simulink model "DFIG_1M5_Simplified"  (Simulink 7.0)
settings: Solver=ode45  SolverMode=SingleTasking  StartTime=0  StopTime=Tstop  FixedStep=0,000005  MaxStep=0.001  RelTol=1e-3  AbsTol=1e-6
InitFcn:
  | DFIG_init_simp
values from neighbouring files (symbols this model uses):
  gearbox = 75.7098    [DFIG_init_simp.m]    (also in DFIG_init_sw.m)
  ki_i = 0.003    [DFIG_init_simp.m]    (also in DFIG_init_sw.m)
  kp_i = 0.00003    (= 3e-05)    [DFIG_init_simp.m]    (also in DFIG_init_sw.m)
  L = 0.6e-3    (= 0.0006)    [DFIG_init_simp.m]    (also in DFIG_init_sw.m)
  R = 35    [DFIG_init_simp.m]    (also in DFIG_init_sw.m)
  TSR_opt = 8    [DFIG_init_simp.m]    (also in DFIG_init_sw.m)
  Tswitch = 0.2    [DFIG_init_simp.m]    (also in DFIG_init_sw.m)
  Vw1 = 10.5    [DFIG_init_simp.m]    (also in DFIG_init_sw.m)
  Vw2 = 8    [DFIG_init_simp.m]    (also in DFIG_init_sw.m)
  zp = 2    [DFIG_init_simp.m]    (also in DFIG_init_sw.m)
undefined symbols (not defined in the file or in its folder): plecsedit
libraries: plecslib x10, plecslib_extras x4, simulink x2

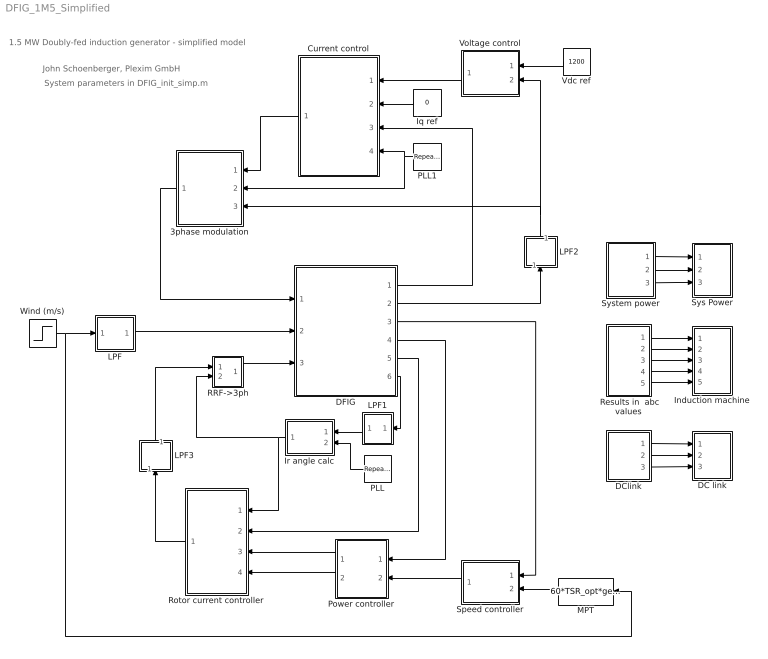
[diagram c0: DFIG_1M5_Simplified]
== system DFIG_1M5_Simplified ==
  note: John Schoenberger, Plexim GmbH
  note: 1.5 MW Doubly-fed induction generator - simplified model
  note: System parameters in DFIG_init_simp.m
  " Results in  abc values" : Subsystem
  3phase modulation : Subsystem  Orientation=left
  Current control : Subsystem  Orientation=left
  DC link : Subsystem  LoadFcn=plecsedit('sl', 300);  StartFcn=plecsedit('sl', 308);  StopFcn=plecsedit('sl', 309);  mask{Settings=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}
      mask init:
      | plecsedit('sl', 315);
  DClink : Subsystem
  DFIG : Subsystem  LoadFcn=plecsedit('sl', 200);  InitFcn=plecsedit('sl', 214);  StartFcn=plecsedit('sl', 208);  StopFcn=plecsedit('sl', 209);
  Induction machine : Subsystem  LoadFcn=plecsedit('sl', 300);  StartFcn=plecsedit('sl', 308);  StopFcn=plecsedit('sl', 309);  mask{Settings=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}
      mask init:
      | plecsedit('sl', 315);
  Iq ref : Constant  Orientation=left  Value=0  OutDataType=sfix(16)  OutScaling=2^0
  Ir angle calc : Subsystem  Orientation=left
  LPF : Subsystem  mask{tau=0.2, y0=Vw1}
      mask prompts: tau "Time constant"; y0 "Initial output"
  LPF1 : Subsystem  Orientation=left  mask(Low-pass filter){tau=1e-4, y0=0}
      mask prompts: tau "Time constant"; y0 "Initial output"
      mask help: First order low pass filter, used in the same way as a memory block to break an algebraic loop. Provides a more deterministic output with a variable-step simulation.
  LPF2 : Subsystem  Orientation=up  mask(Low-pass filter){tau=1e-4, y0=0}
      mask prompts: tau "Time constant"; y0 "Initial output"
      mask help: First order low pass filter, used in the same way as a memory block to break an algebraic loop. Provides a more deterministic output with a variable-step simulation.
  LPF3 : Subsystem  Orientation=up  mask(Low-pass filter){tau=0.5e-4, y0=[0 0]}
      mask prompts: tau "Time constant"; y0 "Initial output"
      mask help: First order low pass filter, used in the same way as a memory block to break an algebraic loop. Provides a more deterministic output with a variable-step simulation.
  MPT : Fcn  Orientation=left  Expr=60*TSR_opt*gearbox*u(1)/(2*pi*R)
  PLL : simulink/Sources/Repeating Sequence  Orientation=left  SystemSampleTime=-1  rep_seq_t=[0 0.02]  rep_seq_y=[-pi/2 3/2*pi]
  PLL1 : simulink/Sources/Repeating Sequence  Orientation=left  SystemSampleTime=-1  rep_seq_t=[0 0.02]  rep_seq_y=[-pi/2 3/2*pi]
  Power controller : Subsystem  Orientation=left
  RRF->3ph : Subsystem  AncestorBlock=plecslib_extras/Transformations/RRF->3ph
  Rotor current controller : Subsystem  Orientation=left
  Speed controller : Subsystem  Orientation=left
  Sys Power : Subsystem  LoadFcn=plecsedit('sl', 300);  StartFcn=plecsedit('sl', 308);  StopFcn=plecsedit('sl', 309);  mask{Settings=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}
      mask init:
      | plecsedit('sl', 315);
  System power : Subsystem
  Vdc ref : Constant  Orientation=left  Value=1200  OutDataType=sfix(16)  OutScaling=2^0
  Voltage control : Subsystem  Orientation=left
  Wind (m/s) : Step  Time=Tswitch  Before=Vw1  After=Vw2  SampleTime=0
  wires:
  RRF->3ph/1(abc) -> DFIG/3(m2)
  DFIG/5(Ir2) -> Rotor current controller/2(Ir2)
  DFIG/6(th r) -> LPF1/1(x)
  Ir angle calc/1(th Ir) -> Rotor current controller/1(theta), RRF->3ph/2(phi)
  " Results in  abc values"/1(Irabc) -> Induction machine/1(1)
  " Results in  abc values"/2(Isabc) -> Induction machine/2(2)
  " Results in  abc values"/3(Vrabc) -> Induction machine/3(3)
  " Results in  abc values"/4(speed) -> Induction machine/4(4)
  " Results in  abc values"/5(Torque) -> Induction machine/5(5)
  DClink/1(Idc in) -> DC link/1(1)
  DClink/2(Vdc) -> DC link/2(2)
  DClink/3(Pdc in) -> DC link/3(3)
  Wind (m/s)/1 -> LPF/1(Vw), MPT/1
  LPF/1(Vw') -> DFIG/2(Vwind)
  Power controller/1(Irq*) -> Rotor current controller/3(Irq*)
  Power controller/2(Ird*) -> Rotor current controller/4(Ird*)
  PLL/1 -> Ir angle calc/2(th 50Hz)
  DFIG/1(Ir1) -> Current control/3(Ir1)
  DFIG/2(Vdc) -> LPF2/1(x)
  System power/1(Stator PQ) -> Sys Power/1(1)
  System power/2(Rotor PQ) -> Sys Power/2(2)
  System power/3(Sys PQ) -> Sys Power/3(3)
  Speed controller/1(P*) -> Power controller/2(P*)
  DFIG/3(rpm) -> Speed controller/1(rpm)
  DFIG/4(P,Q) -> Power controller/1(S)
  MPT/1 -> Speed controller/2(rpm*)
  Voltage control/1(Id*) -> Current control/1(Id*)
  Vdc ref/1 -> Voltage control/1(Vdc*)
  LPF2/1(x') -> 3phase modulation/3(Vdc), Voltage control/2(Vdc)
  Iq ref/1 -> Current control/2(Iq*)
  Current control/1(Vdq*) -> 3phase modulation/1(Vdq*)
  3phase modulation/1(m1) -> DFIG/1(m1)
  PLL1/1 -> 3phase modulation/2(theta), Current control/4(theta)
  LPF1/1(x') -> Ir angle calc/1(th r)
  Rotor current controller/1(Vr dq*) -> LPF3/1(x)
  LPF3/1(x') -> RRF->3ph/1(dq)

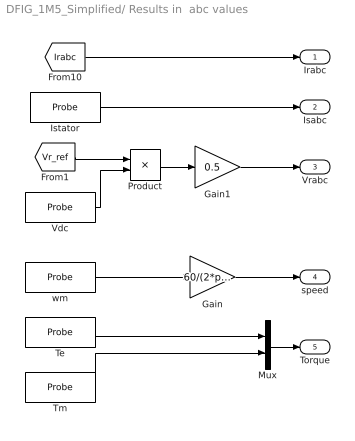
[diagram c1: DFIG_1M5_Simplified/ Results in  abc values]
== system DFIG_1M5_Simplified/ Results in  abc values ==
  Gain : Gain  Gain=60/(2*pi)  ParameterDataType=sfix(16)  ParameterScaling=2^0  OutDataType=sfix(16)  OutScaling=2^0
  Gain1 : Gain  Gain=0.5  ParameterDataType=sfix(16)  ParameterScaling=2^0  OutDataType=sfix(16)  OutScaling=2^0
  Istator : plecslib/Probe  SystemSampleTime=-1  tagno=3
  Mux : Mux  Inputs=2
  Product : Product  OutDataType=sfix(16)  OutScaling=2^0
  Te : plecslib/Probe  SystemSampleTime=-1  tagno=1
  Tm : plecslib/Probe  SystemSampleTime=-1  tagno=5
  Vdc : plecslib/Probe  SystemSampleTime=-1  tagno=4
  wm : plecslib/Probe  SystemSampleTime=-1  tagno=2
  Irabc : Outport
  Isabc : Outport  Port=2
  Vrabc : Outport  Port=3
  speed : Outport  Port=4
  Torque : Outport  Port=5
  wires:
  Gain/1 -> speed/1
  Istator/1 -> Isabc/1
  [Irabc] -> Irabc/1
  Product/1 -> Gain1/1
  Te/1 -> Mux/1
  Tm/1 -> Mux/2
  Mux/1 -> Torque/1
  wm/1 -> Gain/1
  [Vr_ref] -> Product/1
  Vdc/1 -> Product/2
  Gain1/1 -> Vrabc/1

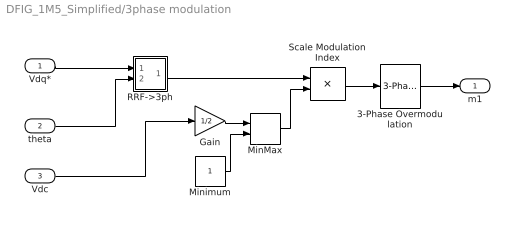
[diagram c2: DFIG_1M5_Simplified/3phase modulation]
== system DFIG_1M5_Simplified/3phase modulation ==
  Vdq* : Inport  OutDataType=sfix(16)  OutScaling=2^0
  theta : Inport  Port=2  OutDataType=sfix(16)  OutScaling=2^0
  Vdc : Inport  Port=3  OutDataType=sfix(16)  OutScaling=2^0
  3-Phase Overmodulation : plecslib_extras/Modulators/3-Phase Overmodulation  SystemSampleTime=-1
  Gain : Gain  Gain=1/2  ParameterDataType=sfix(16)  ParameterScaling=2^0  OutDataType=sfix(16)  OutScaling=2^0
  MinMax : MinMax  Function=max  Inputs=2  OutDataType=sfix(16)  OutScaling=2^0
  Minimum : Constant  OutDataType=sfix(16)  OutScaling=2^0
  RRF->3ph : Subsystem
  Scale Modulation Index : Product  Inputs=*/  OutDataType=sfix(16)  OutScaling=2^0
  m1 : Outport  OutDataType=sfix(16)  OutScaling=2^0
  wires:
  theta/1 -> RRF->3ph/2(phi)
  3-Phase Overmodulation/1 -> m1/1
  Gain/1 -> MinMax/1
  Minimum/1 -> MinMax/2
  MinMax/1 -> Scale Modulation Index/2
  Vdc/1 -> Gain/1
  Scale Modulation Index/1 -> 3-Phase Overmodulation/1
  RRF->3ph/1(abc) -> Scale Modulation Index/1
  Vdq*/1 -> RRF->3ph/1(dq)

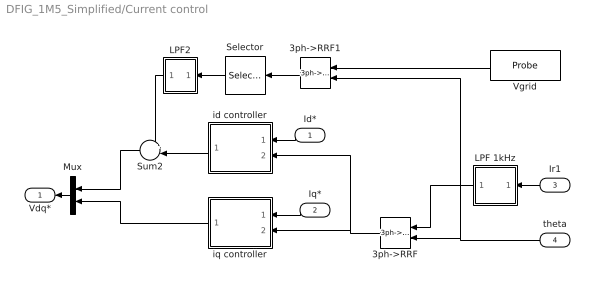
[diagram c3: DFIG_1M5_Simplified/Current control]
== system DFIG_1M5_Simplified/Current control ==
  Id* : Inport  Orientation=left
  Iq* : Inport  Orientation=left  Port=2
  Ir1 : Inport  Orientation=left  Port=3  OutDataType=sfix(16)  OutScaling=2^0
  theta : Inport  Orientation=left  Port=4  OutDataType=sfix(16)  OutScaling=2^0
  3ph->RRF : plecslib_extras/Transformations/3ph->RRF  Orientation=left  SystemSampleTime=-1
  3ph->RRF1 : plecslib_extras/Transformations/3ph->RRF  Orientation=left  SystemSampleTime=-1
  LPF 1kHz : Subsystem  Orientation=left  mask{tau=1.6e-4, y0=0}
      mask prompts: tau "Time constant"; y0 "Initial output"
  LPF2 : Subsystem  Orientation=left  mask(Low-pass filter){tau=1e-4, y0=0}
      mask prompts: tau "Time constant"; y0 "Initial output"
      mask help: First order low pass filter, used in the same way as a memory block to break an algebraic loop. Provides a more deterministic output with a variable-step simulation.
  Mux : Mux  Orientation=left  Inputs=2
  Selector : Selector  Orientation=left  InputPortWidth=2  IndexOptions=Index vector (dialog)  Indices=1  OutputSizes=1
  Sum2 : Sum  Orientation=left  Inputs=+-|  OutDataType=sfix(16)  OutScaling=2^0
  Vgrid : plecslib/Probe  Orientation=left  SystemSampleTime=-1  tagno=6
  id controller : Subsystem  Orientation=left
  iq controller : Subsystem  Orientation=left
  Vdq* : Outport  Orientation=left
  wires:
  iq controller/1(Vq*) -> Mux/2
  Sum2/1 -> Mux/1
  Mux/1 -> Vdq*/1
  Vgrid/1 -> 3ph->RRF1/1
  Ir1/1 -> LPF 1kHz/1(I)
  theta/1 -> 3ph->RRF1/2, 3ph->RRF/2
  Iq*/1 -> iq controller/1(iq ref)
  Id*/1 -> id controller/1(id ref)
  3ph->RRF1/1 -> Selector/1
  3ph->RRF/1 -> id controller/2(i), iq controller/2(i)
  id controller/1(Vd*) -> Sum2/2
  LPF 1kHz/1(Ifilt) -> 3ph->RRF/1
  Selector/1 -> LPF2/1(x)
  LPF2/1(x') -> Sum2/1

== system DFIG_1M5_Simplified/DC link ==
  1 : Inport  OutDataType=sfix(16)  OutScaling=2^0
  2 : Inport  Port=2  OutDataType=sfix(16)  OutScaling=2^0
  3 : Inport  Port=3  OutDataType=sfix(16)  OutScaling=2^0
  " InputMux " : Subsystem
  " S-Function " : S-Function  FunctionName=plecsedit
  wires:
  " InputMux "/1(Out) -> " S-Function "/1
  1/1 -> " InputMux "/1(In1)
  2/1 -> " InputMux "/2(In2)
  3/1 -> " InputMux "/3(In3)

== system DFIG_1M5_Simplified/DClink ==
  DC current from grid converter : plecslib/Probe  SystemSampleTime=-1  tagno=14
  Product : Product  OutDataType=sfix(16)  OutScaling=2^0
  vdc : plecslib/Probe  SystemSampleTime=-1  tagno=15
  Idc in : Outport
  Vdc : Outport  Port=2
  Pdc in : Outport  Port=3
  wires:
  DC current from grid converter/1 -> Idc in/1, Product/1
  vdc/1 -> Vdc/1, Product/2
  Product/1 -> Pdc in/1

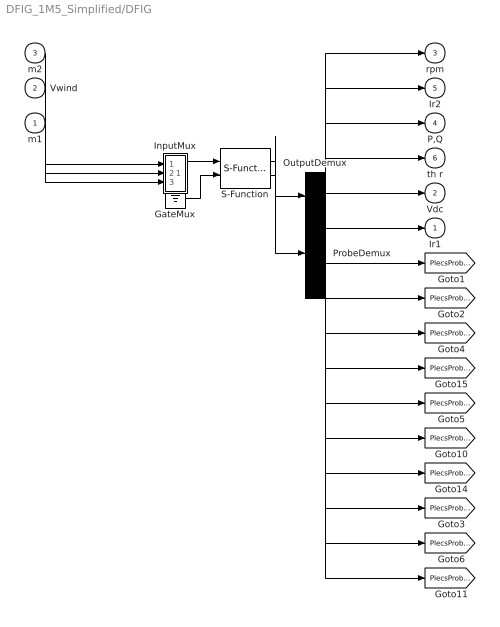
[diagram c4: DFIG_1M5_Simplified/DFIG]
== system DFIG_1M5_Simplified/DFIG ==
  m1 : Inport  PortDimensions=3  OutDataType=sfix(16)  OutScaling=2^0
  Vwind : Inport  Port=2  PortDimensions=1  OutDataType=sfix(16)  OutScaling=2^0
  m2 : Inport  Port=3  PortDimensions=3  OutDataType=sfix(16)  OutScaling=2^0
  " GateMux " : Ground
  " InputMux " : Subsystem
  " OutputDemux " : Demux  Outputs=[ 1 3 2 1 1 3 ]
  " ProbeDemux " : Demux  Outputs=[ 1 1 1 1 1 3 1 3 3 3 ]
  " S-Function " : S-Function  FunctionName=plecsedit
  Ir1 : Outport  PortDimensions=3  OutDataType=sfix(16)  OutScaling=2^0
  Vdc : Outport  Port=2  PortDimensions=1  OutDataType=sfix(16)  OutScaling=2^0
  rpm : Outport  Port=3  PortDimensions=1  OutDataType=sfix(16)  OutScaling=2^0
  P,Q : Outport  Port=4  PortDimensions=2
  Ir2 : Outport  Port=5  PortDimensions=3  OutDataType=sfix(16)  OutScaling=2^0
  th r : Outport  Port=6  PortDimensions=1  OutDataType=sfix(16)  OutScaling=2^0
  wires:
  " S-Function "/2 -> " ProbeDemux "/1
  " GateMux "/1 -> " S-Function "/2
  " InputMux "/1(Out) -> " S-Function "/1
  " S-Function "/1 -> " OutputDemux "/1
  m2/1 -> " InputMux "/1(In1)
  Vwind/1 -> " InputMux "/2(In2)
  m1/1 -> " InputMux "/3(In3)
  " OutputDemux "/1 -> rpm/1
  " OutputDemux "/2 -> Ir2/1
  " OutputDemux "/3 -> P,Q/1
  " OutputDemux "/4 -> th r/1
  " OutputDemux "/5 -> Vdc/1
  " OutputDemux "/6 -> Ir1/1
  " ProbeDemux "/1 -> [PlecsProbe1]
  " ProbeDemux "/2 -> [PlecsProbe2]
  " ProbeDemux "/3 -> [PlecsProbe4]
  " ProbeDemux "/4 -> [PlecsProbe15]
  " ProbeDemux "/5 -> [PlecsProbe5]
  " ProbeDemux "/6 -> [PlecsProbe10]
  " ProbeDemux "/7 -> [PlecsProbe14]
  " ProbeDemux "/8 -> [PlecsProbe3]
  " ProbeDemux "/9 -> [PlecsProbe6]
  " ProbeDemux "/10 -> [PlecsProbe11]

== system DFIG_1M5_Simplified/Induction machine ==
  1 : Inport  OutDataType=sfix(16)  OutScaling=2^0
  2 : Inport  Port=2  OutDataType=sfix(16)  OutScaling=2^0
  3 : Inport  Port=3  OutDataType=sfix(16)  OutScaling=2^0
  4 : Inport  Port=4  OutDataType=sfix(16)  OutScaling=2^0
  5 : Inport  Port=5  OutDataType=sfix(16)  OutScaling=2^0
  " InputMux " : Subsystem
  " S-Function " : S-Function  FunctionName=plecsedit
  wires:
  " InputMux "/1(Out) -> " S-Function "/1
  1/1 -> " InputMux "/1(In1)
  2/1 -> " InputMux "/2(In2)
  3/1 -> " InputMux "/3(In3)
  4/1 -> " InputMux "/4(In4)
  5/1 -> " InputMux "/5(In5)

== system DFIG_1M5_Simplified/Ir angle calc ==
  th r : Inport  OutDataType=sfix(16)  OutScaling=2^0
  th 50Hz : Inport  Port=2  OutDataType=sfix(16)  OutScaling=2^0
  Gain : Gain  Gain=zp  ParameterDataType=sfix(16)  ParameterScaling=2^0  OutDataType=sfix(16)  OutScaling=2^0
  Sum1 : Sum  Inputs=+-  OutDataType=sfix(16)  OutScaling=2^0
  th Ir : Outport
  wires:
  th r/1 -> Gain/1
  th 50Hz/1 -> Sum1/1
  Sum1/1 -> th Ir/1
  Gain/1 -> Sum1/2

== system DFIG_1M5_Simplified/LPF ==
  Vw : Inport  OutDataType=sfix(16)  OutScaling=2^0
  Gain : Gain  Gain=1/tau  ParameterDataType=sfix(16)  ParameterScaling=2^0  OutDataType=sfix(16)  OutScaling=2^0
  Integrator : Integrator  InitialCondition=y0
  Subtract : Sum  Inputs=+-  OutDataType=sfix(16)  OutScaling=2^-10
  Vw' : Outport  OutDataType=sfix(16)  OutScaling=2^0
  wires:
  Integrator/1 -> Vw'/1, Subtract/2
  Vw/1 -> Subtract/1
  Subtract/1 -> Gain/1
  Gain/1 -> Integrator/1

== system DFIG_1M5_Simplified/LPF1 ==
  x : Inport  OutDataType=sfix(16)  OutScaling=2^0
  Gain : Gain  Gain=1/tau  ParameterDataType=sfix(16)  ParameterScaling=2^0  OutDataType=sfix(16)  OutScaling=2^0
  Integrator : Integrator  InitialCondition=y0
  Subtract : Sum  Inputs=+-  OutDataType=sfix(16)  OutScaling=2^-10
  x' : Outport  OutDataType=sfix(16)  OutScaling=2^0
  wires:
  Integrator/1 -> x'/1, Subtract/2
  x/1 -> Subtract/1
  Subtract/1 -> Gain/1
  Gain/1 -> Integrator/1

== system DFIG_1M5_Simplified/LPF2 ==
  x : Inport  OutDataType=sfix(16)  OutScaling=2^0
  Gain : Gain  Gain=1/tau  ParameterDataType=sfix(16)  ParameterScaling=2^0  OutDataType=sfix(16)  OutScaling=2^0
  Integrator : Integrator  InitialCondition=y0
  Subtract : Sum  Inputs=+-  OutDataType=sfix(16)  OutScaling=2^-10
  x' : Outport  OutDataType=sfix(16)  OutScaling=2^0
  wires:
  Integrator/1 -> x'/1, Subtract/2
  x/1 -> Subtract/1
  Subtract/1 -> Gain/1
  Gain/1 -> Integrator/1

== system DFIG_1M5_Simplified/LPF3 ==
  x : Inport  OutDataType=sfix(16)  OutScaling=2^0
  Gain : Gain  Gain=1/tau  ParameterDataType=sfix(16)  ParameterScaling=2^0  OutDataType=sfix(16)  OutScaling=2^0
  Integrator : Integrator  InitialCondition=y0
  Subtract : Sum  Inputs=+-  OutDataType=sfix(16)  OutScaling=2^-10
  x' : Outport  OutDataType=sfix(16)  OutScaling=2^0
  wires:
  Integrator/1 -> x'/1, Subtract/2
  x/1 -> Subtract/1
  Subtract/1 -> Gain/1
  Gain/1 -> Integrator/1

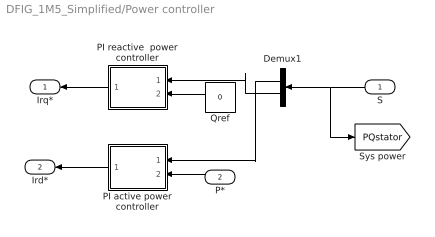
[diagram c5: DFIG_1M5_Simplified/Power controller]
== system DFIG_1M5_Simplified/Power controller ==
  S : Inport  Orientation=left  OutDataType=sfix(16)  OutScaling=2^0
  P* : Inport  Orientation=left  Port=2  OutDataType=sfix(16)  OutScaling=2^0
  Demux1 : Demux  Orientation=left  Outputs=2
  PI active power controller : Subsystem  Orientation=left
  PI reactive  power controller : Subsystem  Orientation=left
  Qref : Constant  Orientation=left  Value=0  OutDataType=sfix(16)  OutScaling=2^0
  Irq* : Outport  Orientation=left  OutDataType=sfix(16)  OutScaling=2^0
  Ird* : Outport  Orientation=left  Port=2  OutDataType=sfix(16)  OutScaling=2^0
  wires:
  Qref/1 -> PI reactive  power controller/2(Qref)
  PI reactive  power controller/1(Irqref) -> Irq*/1
  PI active power controller/1(Irdref) -> Ird*/1
  P*/1 -> PI active power controller/2(Pref)
  S/1 -> Demux1/1, [PQstator]
  Demux1/1 -> PI active power controller/1(P)
  Demux1/2 -> PI reactive  power controller/1(Q)

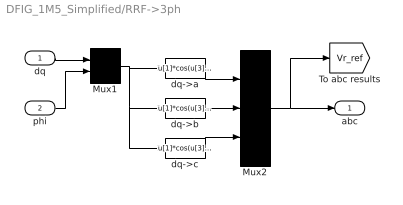
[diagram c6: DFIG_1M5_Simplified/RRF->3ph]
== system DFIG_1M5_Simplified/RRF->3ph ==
  dq : Inport  PortDimensions=2
  phi : Inport  Port=2  PortDimensions=1
  Mux1 : Mux  Inputs=2
  Mux2 : Mux  Inputs=3
  dq->a : Fcn  Expr=u[1]*cos(u[3])-u[2]*sin(u[3])
  dq->b : Fcn  Expr=u[1]*cos(u[3]-2*pi/3)-u[2]*sin(u[3]-2*pi/3)
  dq->c : Fcn  Expr=u[1]*cos(u[3]+2*pi/3)-u[2]*sin(u[3]+2*pi/3)
  abc : Outport
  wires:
  phi/1 -> Mux1/2
  dq/1 -> Mux1/1
  Mux1/1 -> dq->a/1, dq->b/1, dq->c/1
  dq->a/1 -> Mux2/1
  dq->b/1 -> Mux2/2
  Mux2/1 -> abc/1, [Vr_ref]
  dq->c/1 -> Mux2/3

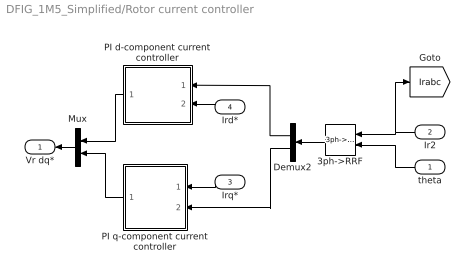
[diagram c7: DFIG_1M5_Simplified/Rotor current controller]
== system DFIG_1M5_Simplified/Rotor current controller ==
  theta : Inport  Orientation=left  OutDataType=sfix(16)  OutScaling=2^0
  Ir2 : Inport  Orientation=left  Port=2  OutDataType=sfix(16)  OutScaling=2^0
  Irq* : Inport  Orientation=left  Port=3  OutDataType=sfix(16)  OutScaling=2^0
  Ird* : Inport  Orientation=left  Port=4  OutDataType=sfix(16)  OutScaling=2^0
  3ph->RRF : plecslib_extras/Transformations/3ph->RRF  Orientation=left  SystemSampleTime=-1
  Demux2 : Demux  Orientation=left  Outputs=2
  Mux : Mux  Orientation=left  Inputs=2
  PI d-component current controller : Subsystem  Orientation=left
  PI q-component current controller : Subsystem  Orientation=left
  Vr dq* : Outport  Orientation=left  OutDataType=sfix(16)  OutScaling=2^0
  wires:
  Irq*/1 -> PI q-component current controller/1(Irqref)
  Ird*/1 -> PI d-component current controller/2(Irdref)
  Mux/1 -> Vr dq*/1
  PI d-component current controller/1(Vrd) -> Mux/1
  PI q-component current controller/1(Vrq) -> Mux/2
  3ph->RRF/1 -> Demux2/1
  Ir2/1 -> 3ph->RRF/1, [Irabc]
  theta/1 -> 3ph->RRF/2
  Demux2/1 -> PI d-component current controller/1(Ird)
  Demux2/2 -> PI q-component current controller/2(Irq)

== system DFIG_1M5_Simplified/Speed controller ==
  rpm : Inport  Orientation=left  OutDataType=sfix(16)  OutScaling=2^0
  rpm* : Inport  Orientation=left  Port=2  OutDataType=sfix(16)  OutScaling=2^0
  Integrator : Integrator  Orientation=left  UpperSaturationLimit=5000  LowerSaturationLimit=-5000
  Ki : Gain  Orientation=left  Gain=1500  ParameterDataType=sfix(16)  ParameterScaling=2^0  OutDataType=sfix(16)  OutScaling=2^0
  Kp : Gain  Orientation=left  Gain=750  ParameterDataType=sfix(16)  ParameterScaling=2^0  OutDataType=sfix(16)  OutScaling=2^0
  Sum1 : Sum  Orientation=left  OutDataType=sfix(16)  OutScaling=2^0
  Sum3 : Sum  Orientation=left  Inputs=+-  OutDataType=sfix(16)  OutScaling=2^0
  P* : Outport  Orientation=left
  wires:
  Sum3/1 -> Kp/1, Ki/1
  Ki/1 -> Integrator/1
  Kp/1 -> Sum1/1
  Sum1/1 -> P*/1
  Integrator/1 -> Sum1/2
  rpm*/1 -> Sum3/1
  rpm/1 -> Sum3/2

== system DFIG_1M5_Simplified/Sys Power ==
  1 : Inport  OutDataType=sfix(16)  OutScaling=2^0
  2 : Inport  Port=2  OutDataType=sfix(16)  OutScaling=2^0
  3 : Inport  Port=3  OutDataType=sfix(16)  OutScaling=2^0
  " InputMux " : Subsystem
  " S-Function " : S-Function  FunctionName=plecsedit
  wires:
  " InputMux "/1(Out) -> " S-Function "/1
  1/1 -> " InputMux "/1(In1)
  2/1 -> " InputMux "/2(In2)
  3/1 -> " InputMux "/3(In3)

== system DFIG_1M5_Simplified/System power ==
  3 phase  P & Q1 : Subsystem  DialogController=PMDialogs.PMDefaultMaskDlg
  Rotor current : plecslib/Probe  SystemSampleTime=-1  tagno=10
  Sum of Elements : Sum  OutDataType=sfix(16)  OutScaling=2^-10
  Sys voltage : plecslib/Probe  SystemSampleTime=-1  tagno=11
  Stator PQ : Outport
  Rotor PQ : Outport  Port=2
  Sys PQ : Outport  Port=3
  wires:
  3 phase  P & Q1/1(PQ) -> Rotor PQ/1, Sum of Elements/2
  Sys voltage/1 -> 3 phase  P & Q1/1(Vabc)
  Rotor current/1 -> 3 phase  P & Q1/2(Iabc)
  [PQstator] -> Stator PQ/1, Sum of Elements/1
  Sum of Elements/1 -> Sys PQ/1

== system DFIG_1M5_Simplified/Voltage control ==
  Vdc* : Inport  Orientation=left  PortDimensions=1  OutDataType=sfix(16)  OutScaling=2^0
  Vdc : Inport  Orientation=left  Port=2  PortDimensions=1  OutDataType=sfix(16)  OutScaling=2^0
  I : Gain  Orientation=left  Gain=20  ParameterDataType=sfix(16)  ParameterScaling=2^0  OutDataType=sfix(16)  OutScaling=2^0
  Integrator : Integrator  Orientation=left
  P : Gain  Orientation=left  Gain=2  ParameterDataType=sfix(16)  ParameterScaling=2^0  OutDataType=sfix(16)  OutScaling=2^0
  Sum1 : Sum  Orientation=left  OutDataType=sfix(16)  OutScaling=2^0
  Sum2 : Sum  Orientation=left  Inputs=+-  OutDataType=sfix(16)  OutScaling=2^0
  Id* : Outport  Orientation=left  OutDataType=sfix(16)  OutScaling=2^0
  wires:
  P/1 -> Sum1/1
  I/1 -> Integrator/1
  Sum1/1 -> Id*/1
  Sum2/1 -> P/1, I/1
  Vdc*/1 -> Sum2/1
  Vdc/1 -> Sum2/2
  Integrator/1 -> Sum1/2

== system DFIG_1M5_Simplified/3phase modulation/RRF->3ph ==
  dq : Inport  PortDimensions=2  OutDataType=sfix(16)  OutScaling=2^0
  phi : Inport  Port=2  PortDimensions=1  OutDataType=sfix(16)  OutScaling=2^0
  Mux1 : Mux  Inputs=2
  Mux2 : Mux  Inputs=3
  dq->a : Fcn  Expr=u[1]*cos(u[3])-u[2]*sin(u[3])
  dq->b : Fcn  Expr=u[1]*cos(u[3]-2*pi/3)-u[2]*sin(u[3]-2*pi/3)
  dq->c : Fcn  Expr=u[1]*cos(u[3]+2*pi/3)-u[2]*sin(u[3]+2*pi/3)
  abc : Outport  OutDataType=sfix(16)  OutScaling=2^0
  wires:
  dq->c/1 -> Mux2/3
  Mux2/1 -> abc/1
  dq->b/1 -> Mux2/2
  dq->a/1 -> Mux2/1
  Mux1/1 -> dq->c/1, dq->b/1, dq->a/1
  dq/1 -> Mux1/1
  phi/1 -> Mux1/2

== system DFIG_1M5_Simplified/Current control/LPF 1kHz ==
  I : Inport  OutDataType=sfix(16)  OutScaling=2^0
  Gain : Gain  Gain=1/tau  ParameterDataType=sfix(16)  ParameterScaling=2^0  OutDataType=sfix(16)  OutScaling=2^0
  Integrator : Integrator  InitialCondition=y0
  Subtract : Sum  Inputs=+-  OutDataType=sfix(16)  OutScaling=2^-10
  Ifilt : Outport  OutDataType=sfix(16)  OutScaling=2^0
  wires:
  Gain/1 -> Integrator/1
  Subtract/1 -> Gain/1
  I/1 -> Subtract/1
  Integrator/1 -> Subtract/2, Ifilt/1

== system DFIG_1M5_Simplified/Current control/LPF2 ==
  x : Inport  OutDataType=sfix(16)  OutScaling=2^0
  Gain : Gain  Gain=1/tau  ParameterDataType=sfix(16)  ParameterScaling=2^0  OutDataType=sfix(16)  OutScaling=2^0
  Integrator : Integrator  InitialCondition=y0
  Subtract : Sum  Inputs=+-  OutDataType=sfix(16)  OutScaling=2^-10
  x' : Outport  OutDataType=sfix(16)  OutScaling=2^0
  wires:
  Gain/1 -> Integrator/1
  Subtract/1 -> Gain/1
  x/1 -> Subtract/1
  Integrator/1 -> Subtract/2, x'/1

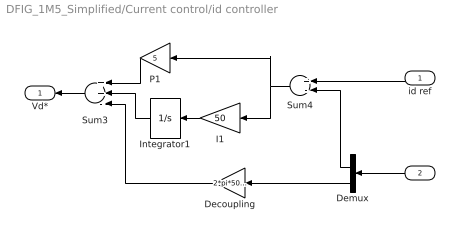
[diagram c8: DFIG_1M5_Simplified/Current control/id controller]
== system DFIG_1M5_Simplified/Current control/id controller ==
  id ref : Inport  Orientation=left  OutDataType=sfix(16)  OutScaling=2^0
  i : Inport  Orientation=left  Port=2  PortDimensions=2  OutDataType=sfix(16)  OutScaling=2^0
  Decoupling : Gain  Orientation=left  Gain=2*pi*50*L  Multiplication=Matrix(K*u)  ParameterDataType=sfix(16)  ParameterScaling=2^0  OutDataType=sfix(16)  OutScaling=2^0
  Demux : Demux  Orientation=left  Outputs=2
  I1 : Gain  Orientation=left  Gain=50  ParameterDataType=sfix(16)  ParameterScaling=2^0  OutDataType=sfix(16)  OutScaling=2^0
  Integrator1 : Integrator  Orientation=left
  P1 : Gain  Orientation=left  Gain=5  ParameterDataType=sfix(16)  ParameterScaling=2^0  OutDataType=sfix(16)  OutScaling=2^0
  Sum3 : Sum  Orientation=left  Inputs=++-  OutDataType=sfix(16)  OutScaling=2^0
  Sum4 : Sum  Orientation=left  Inputs=+-  OutDataType=sfix(16)  OutScaling=2^0
  Vd* : Outport  Orientation=left  OutDataType=sfix(16)  OutScaling=2^0
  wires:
  P1/1 -> Sum3/1
  I1/1 -> Integrator1/1
  Sum4/1 -> I1/1, P1/1
  Integrator1/1 -> Sum3/2
  id ref/1 -> Sum4/1
  Decoupling/1 -> Sum3/3
  Demux/1 -> Sum4/2
  Demux/2 -> Decoupling/1
  i/1 -> Demux/1
  Sum3/1 -> Vd*/1

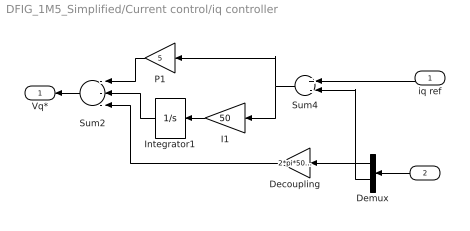
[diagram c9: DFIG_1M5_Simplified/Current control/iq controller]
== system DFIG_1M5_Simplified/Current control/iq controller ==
  iq ref : Inport  Orientation=left  OutDataType=sfix(16)  OutScaling=2^0
  i : Inport  Orientation=left  Port=2  PortDimensions=2  OutDataType=sfix(16)  OutScaling=2^0
  Decoupling : Gain  Orientation=left  Gain=2*pi*50*L  Multiplication=Matrix(K*u)  ParameterDataType=sfix(16)  ParameterScaling=2^0  OutDataType=sfix(16)  OutScaling=2^0
  Demux : Demux  Orientation=left  Outputs=2
  I1 : Gain  Orientation=left  Gain=50  ParameterDataType=sfix(16)  ParameterScaling=2^0  OutDataType=sfix(16)  OutScaling=2^0
  Integrator1 : Integrator  Orientation=left
  P1 : Gain  Orientation=left  Gain=5  ParameterDataType=sfix(16)  ParameterScaling=2^0  OutDataType=sfix(16)  OutScaling=2^0
  Sum2 : Sum  Orientation=left  Inputs=---  OutDataType=sfix(16)  OutScaling=2^0
  Sum4 : Sum  Orientation=left  Inputs=+-  OutDataType=sfix(16)  OutScaling=2^0
  Vq* : Outport  Orientation=left  OutDataType=sfix(16)  OutScaling=2^0
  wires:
  I1/1 -> Integrator1/1
  Sum4/1 -> P1/1, I1/1
  Integrator1/1 -> Sum2/2
  iq ref/1 -> Sum4/1
  Decoupling/1 -> Sum2/3
  i/1 -> Demux/1
  P1/1 -> Sum2/1
  Sum2/1 -> Vq*/1
  Demux/2 -> Sum4/2
  Demux/1 -> Decoupling/1

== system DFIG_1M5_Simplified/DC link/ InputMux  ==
  In1 : Inport  OutDataType=sfix(16)  OutScaling=2^0
  In2 : Inport  Port=2  OutDataType=sfix(16)  OutScaling=2^0
  In3 : Inport  Port=3  OutDataType=sfix(16)  OutScaling=2^0
  Convert1 : DataTypeConversion  OutDataType=sfix(16)  OutScaling=2^0
  Convert2 : DataTypeConversion  OutDataType=sfix(16)  OutScaling=2^0
  Convert3 : DataTypeConversion  OutDataType=sfix(16)  OutScaling=2^0
  Mux : Mux  Inputs=3
  Out : Outport  OutDataType=sfix(16)  OutScaling=2^0
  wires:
  Mux/1 -> Out/1
  In1/1 -> Convert1/1
  In2/1 -> Convert2/1
  In3/1 -> Convert3/1
  Convert1/1 -> Mux/1
  Convert2/1 -> Mux/2
  Convert3/1 -> Mux/3

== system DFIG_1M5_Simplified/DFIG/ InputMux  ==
  In1 : Inport  OutDataType=sfix(16)  OutScaling=2^0
  In2 : Inport  Port=2  OutDataType=sfix(16)  OutScaling=2^0
  In3 : Inport  Port=3  OutDataType=sfix(16)  OutScaling=2^0
  Convert1 : DataTypeConversion  OutDataType=sfix(16)  OutScaling=2^0
  Convert2 : DataTypeConversion  OutDataType=sfix(16)  OutScaling=2^0
  Convert3 : DataTypeConversion  OutDataType=sfix(16)  OutScaling=2^0
  Mux : Mux  Inputs=[ 3 1 3 ]
  Out : Outport  OutDataType=sfix(16)  OutScaling=2^0
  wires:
  Mux/1 -> Out/1
  In1/1 -> Convert1/1
  In2/1 -> Convert2/1
  In3/1 -> Convert3/1
  Convert1/1 -> Mux/1
  Convert2/1 -> Mux/2
  Convert3/1 -> Mux/3

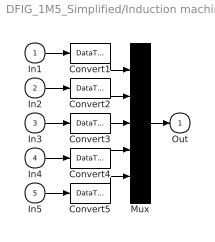
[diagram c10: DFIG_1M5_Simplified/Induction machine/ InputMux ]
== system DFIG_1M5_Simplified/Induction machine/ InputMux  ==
  In1 : Inport  OutDataType=sfix(16)  OutScaling=2^0
  In2 : Inport  Port=2  OutDataType=sfix(16)  OutScaling=2^0
  In3 : Inport  Port=3  OutDataType=sfix(16)  OutScaling=2^0
  In4 : Inport  Port=4  OutDataType=sfix(16)  OutScaling=2^0
  In5 : Inport  Port=5  OutDataType=sfix(16)  OutScaling=2^0
  Convert{1..5} (5 alike) : DataTypeConversion  OutDataType=sfix(16)  OutScaling=2^0
  Mux : Mux  Inputs=5
  Out : Outport  OutDataType=sfix(16)  OutScaling=2^0
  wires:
  Mux/1 -> Out/1
  In1/1 -> Convert1/1
  In2/1 -> Convert2/1
  In3/1 -> Convert3/1
  In4/1 -> Convert4/1
  In5/1 -> Convert5/1
  Convert1/1 -> Mux/1
  Convert2/1 -> Mux/2
  Convert3/1 -> Mux/3
  Convert4/1 -> Mux/4
  Convert5/1 -> Mux/5

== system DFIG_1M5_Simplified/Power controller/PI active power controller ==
  P : Inport  Orientation=left  OutDataType=sfix(16)  OutScaling=2^0
  Pref : Inport  Orientation=left  Port=2  OutDataType=sfix(16)  OutScaling=2^0
  Gain : Gain  Orientation=left  Gain=0.0002  ParameterDataType=sfix(16)  ParameterScaling=2^0  OutDataType=sfix(16)  OutScaling=2^0
  Gain1 : Gain  Orientation=left  Gain=0.05  ParameterDataType=sfix(16)  ParameterScaling=2^0  OutDataType=sfix(16)  OutScaling=2^0
  Integrator2 : Integrator  Orientation=left
  Sum2 : Sum  Orientation=left  Inputs=|+-  OutDataType=sfix(16)  OutScaling=2^0
  Sum3 : Sum  Orientation=left  Inputs=+-  OutDataType=sfix(16)  OutScaling=2^0
  Irdref : Outport  Orientation=left
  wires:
  Integrator2/1 -> Sum2/2
  Sum3/1 -> Gain/1, Gain1/1
  P/1 -> Sum3/2
  Pref/1 -> Sum3/1
  Sum2/1 -> Irdref/1
  Gain/1 -> Sum2/1
  Gain1/1 -> Integrator2/1

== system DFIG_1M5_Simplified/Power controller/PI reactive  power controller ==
  Q : Inport  Orientation=left  OutDataType=sfix(16)  OutScaling=2^0
  Qref : Inport  Orientation=left  Port=2  OutDataType=sfix(16)  OutScaling=2^0
  -1/(sqrt(3)*Vpp) : Gain  Orientation=left  Gain=0.0002  ParameterDataType=sfix(16)  ParameterScaling=2^0  OutDataType=sfix(16)  OutScaling=2^0
  Gain6 : Gain  Orientation=left  Gain=0.005  ParameterDataType=sfix(16)  ParameterScaling=2^0  OutDataType=sfix(16)  OutScaling=2^0
  Integrator2 : Integrator  Orientation=left
  Sum2 : Sum  Orientation=left  Inputs=|++  OutDataType=sfix(16)  OutScaling=2^0
  Sum3 : Sum  Orientation=left  Inputs=+-  OutDataType=sfix(16)  OutScaling=2^0
  Irqref : Outport  Orientation=left
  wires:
  Gain6/1 -> Integrator2/1
  Sum3/1 -> -1/(sqrt(3)*Vpp)/1, Gain6/1
  Q/1 -> Sum3/2
  Qref/1 -> Sum3/1
  Sum2/1 -> Irqref/1
  Integrator2/1 -> Sum2/2
  -1/(sqrt(3)*Vpp)/1 -> Sum2/1

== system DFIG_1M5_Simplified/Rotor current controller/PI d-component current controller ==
  Ird : Inport  Orientation=left  OutDataType=sfix(16)  OutScaling=2^0
  Irdref : Inport  Orientation=left  Port=2  OutDataType=sfix(16)  OutScaling=2^0
  Gain3 : Gain  Orientation=left  Gain=kp_i  ParameterDataType=sfix(16)  ParameterScaling=2^0  OutDataType=sfix(16)  OutScaling=2^0
  Gain4 : Gain  Orientation=left  Gain=ki_i  ParameterDataType=sfix(16)  ParameterScaling=2^0  OutDataType=sfix(16)  OutScaling=2^0
  Integrator1 : Integrator  Orientation=left
  Sum4 : Sum  Orientation=left  Inputs=+-  OutDataType=sfix(16)  OutScaling=2^0
  Sum5 : Sum  Orientation=left  Inputs=|++  OutDataType=sfix(16)  OutScaling=2^0
  Vrd : Outport  Orientation=left
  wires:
  Gain3/1 -> Sum5/1
  Gain4/1 -> Integrator1/1
  Sum4/1 -> Gain3/1, Gain4/1
  Sum5/1 -> Vrd/1
  Irdref/1 -> Sum4/1
  Ird/1 -> Sum4/2
  Integrator1/1 -> Sum5/2

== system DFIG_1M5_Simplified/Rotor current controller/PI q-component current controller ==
  Irqref : Inport  Orientation=left  OutDataType=sfix(16)  OutScaling=2^0
  Irq : Inport  Orientation=left  Port=2  OutDataType=sfix(16)  OutScaling=2^0
  Integrator1 : Integrator  Orientation=left
  Ki : Gain  Orientation=left  Gain=ki_i  ParameterDataType=sfix(16)  ParameterScaling=2^0  OutDataType=sfix(16)  OutScaling=2^0
  Kp : Gain  Orientation=left  Gain=kp_i  ParameterDataType=sfix(16)  ParameterScaling=2^0  OutDataType=sfix(16)  OutScaling=2^0
  Sum : Sum  Orientation=left  OutDataType=sfix(16)  OutScaling=2^0
  Sum1 : Sum  Orientation=left  Inputs=+-  OutDataType=sfix(16)  OutScaling=2^0
  Vrq : Outport  Orientation=left
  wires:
  Kp/1 -> Sum/1
  Ki/1 -> Integrator1/1
  Integrator1/1 -> Sum/2
  Irqref/1 -> Sum1/1
  Irq/1 -> Sum1/2
  Sum/1 -> Vrq/1
  Sum1/1 -> Kp/1, Ki/1

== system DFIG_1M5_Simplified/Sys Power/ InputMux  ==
  In1 : Inport  OutDataType=sfix(16)  OutScaling=2^0
  In2 : Inport  Port=2  OutDataType=sfix(16)  OutScaling=2^0
  In3 : Inport  Port=3  OutDataType=sfix(16)  OutScaling=2^0
  Convert1 : DataTypeConversion  OutDataType=sfix(16)  OutScaling=2^0
  Convert2 : DataTypeConversion  OutDataType=sfix(16)  OutScaling=2^0
  Convert3 : DataTypeConversion  OutDataType=sfix(16)  OutScaling=2^0
  Mux : Mux  Inputs=3
  Out : Outport  OutDataType=sfix(16)  OutScaling=2^0
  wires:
  Mux/1 -> Out/1
  In1/1 -> Convert1/1
  In2/1 -> Convert2/1
  In3/1 -> Convert3/1
  Convert1/1 -> Mux/1
  Convert2/1 -> Mux/2
  Convert3/1 -> Mux/3

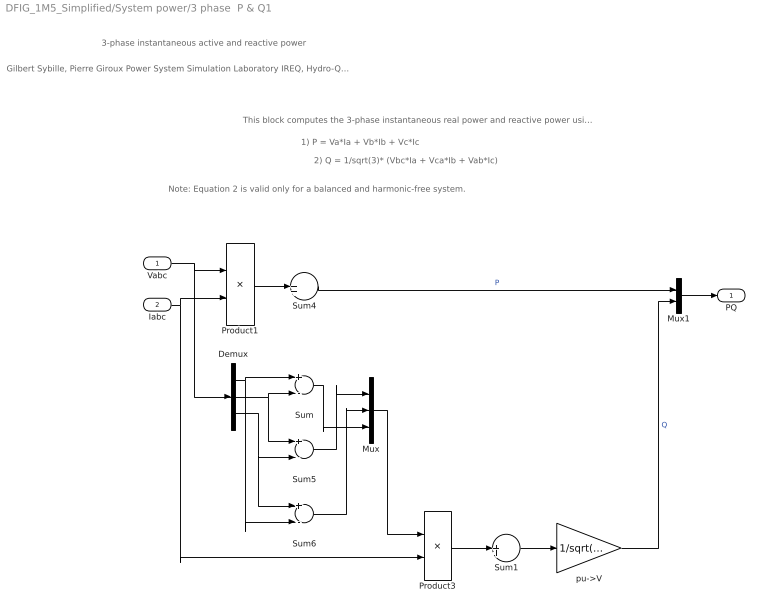
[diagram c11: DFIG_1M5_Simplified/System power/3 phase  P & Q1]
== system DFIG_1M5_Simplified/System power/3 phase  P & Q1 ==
  note: 1) P = Va*Ia + Vb*Ib + Vc*Ic
  note: 2) Q = 1/sqrt(3)* (Vbc*Ia + Vca*Ib + Vab*Ic)
  note: This block computes the 3-phase instantaneous real power and reactive power using the following equations:
  note: Note: Equation 2 is valid only for a balanced and harmonic-free system.
  note: 3-phase instantaneous active and reactive power
  note: Gilbert Sybille, Pierre Giroux Power System Simulation Laboratory IREQ, Hydro-Quebc
  Vabc : Inport  PortDimensions=3  OutDataType=sfix(16)  OutScaling=2^0
  Iabc : Inport  Port=2  PortDimensions=3  OutDataType=sfix(16)  OutScaling=2^0
  Demux : Demux  Outputs=3
  Mux : Mux  Inputs=3
  Mux1 : Mux  Inputs=2
  Product1 : Product  OutDataType=sfix(16)  OutScaling=2^0
  Product3 : Product  OutDataType=sfix(16)  OutScaling=2^0
  Sum : Sum  Inputs=+-  OutDataType=sfix(16)  OutScaling=2^0
  Sum1 : Sum  Inputs=1  OutDataType=sfix(16)  OutScaling=2^0
  Sum4 : Sum  Inputs=1  OutDataType=sfix(16)  OutScaling=2^0
  Sum5 : Sum  Inputs=+-  OutDataType=sfix(16)  OutScaling=2^0
  Sum6 : Sum  Inputs=+-  OutDataType=sfix(16)  OutScaling=2^0
  pu->V : Gain  Gain=1/sqrt(3)  ParameterDataType=sfix(16)  ParameterScaling=2^0  OutDataType=sfix(16)  OutScaling=2^0
  PQ : Outport  OutDataType=sfix(16)  OutScaling=2^0
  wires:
  Sum1/1 -> pu->V/1
  Product3/1 -> Sum1/1
  Product1/1 -> Sum4/1
  Vabc/1 -> Product1/1, Demux/1
  Iabc/1 -> Product1/2, Product3/2
  Sum4/1 -> Mux1/1  "P"
  Demux/1 -> Sum/1, Sum6/2
  Demux/2 -> Sum/2, Sum5/1
  Demux/3 -> Sum5/2, Sum6/1
  Sum/1 -> Mux/3
  Sum5/1 -> Mux/1
  Sum6/1 -> Mux/2
  Mux/1 -> Product3/1
  pu->V/1 -> Mux1/2  "Q"
  Mux1/1 -> PQ/1
